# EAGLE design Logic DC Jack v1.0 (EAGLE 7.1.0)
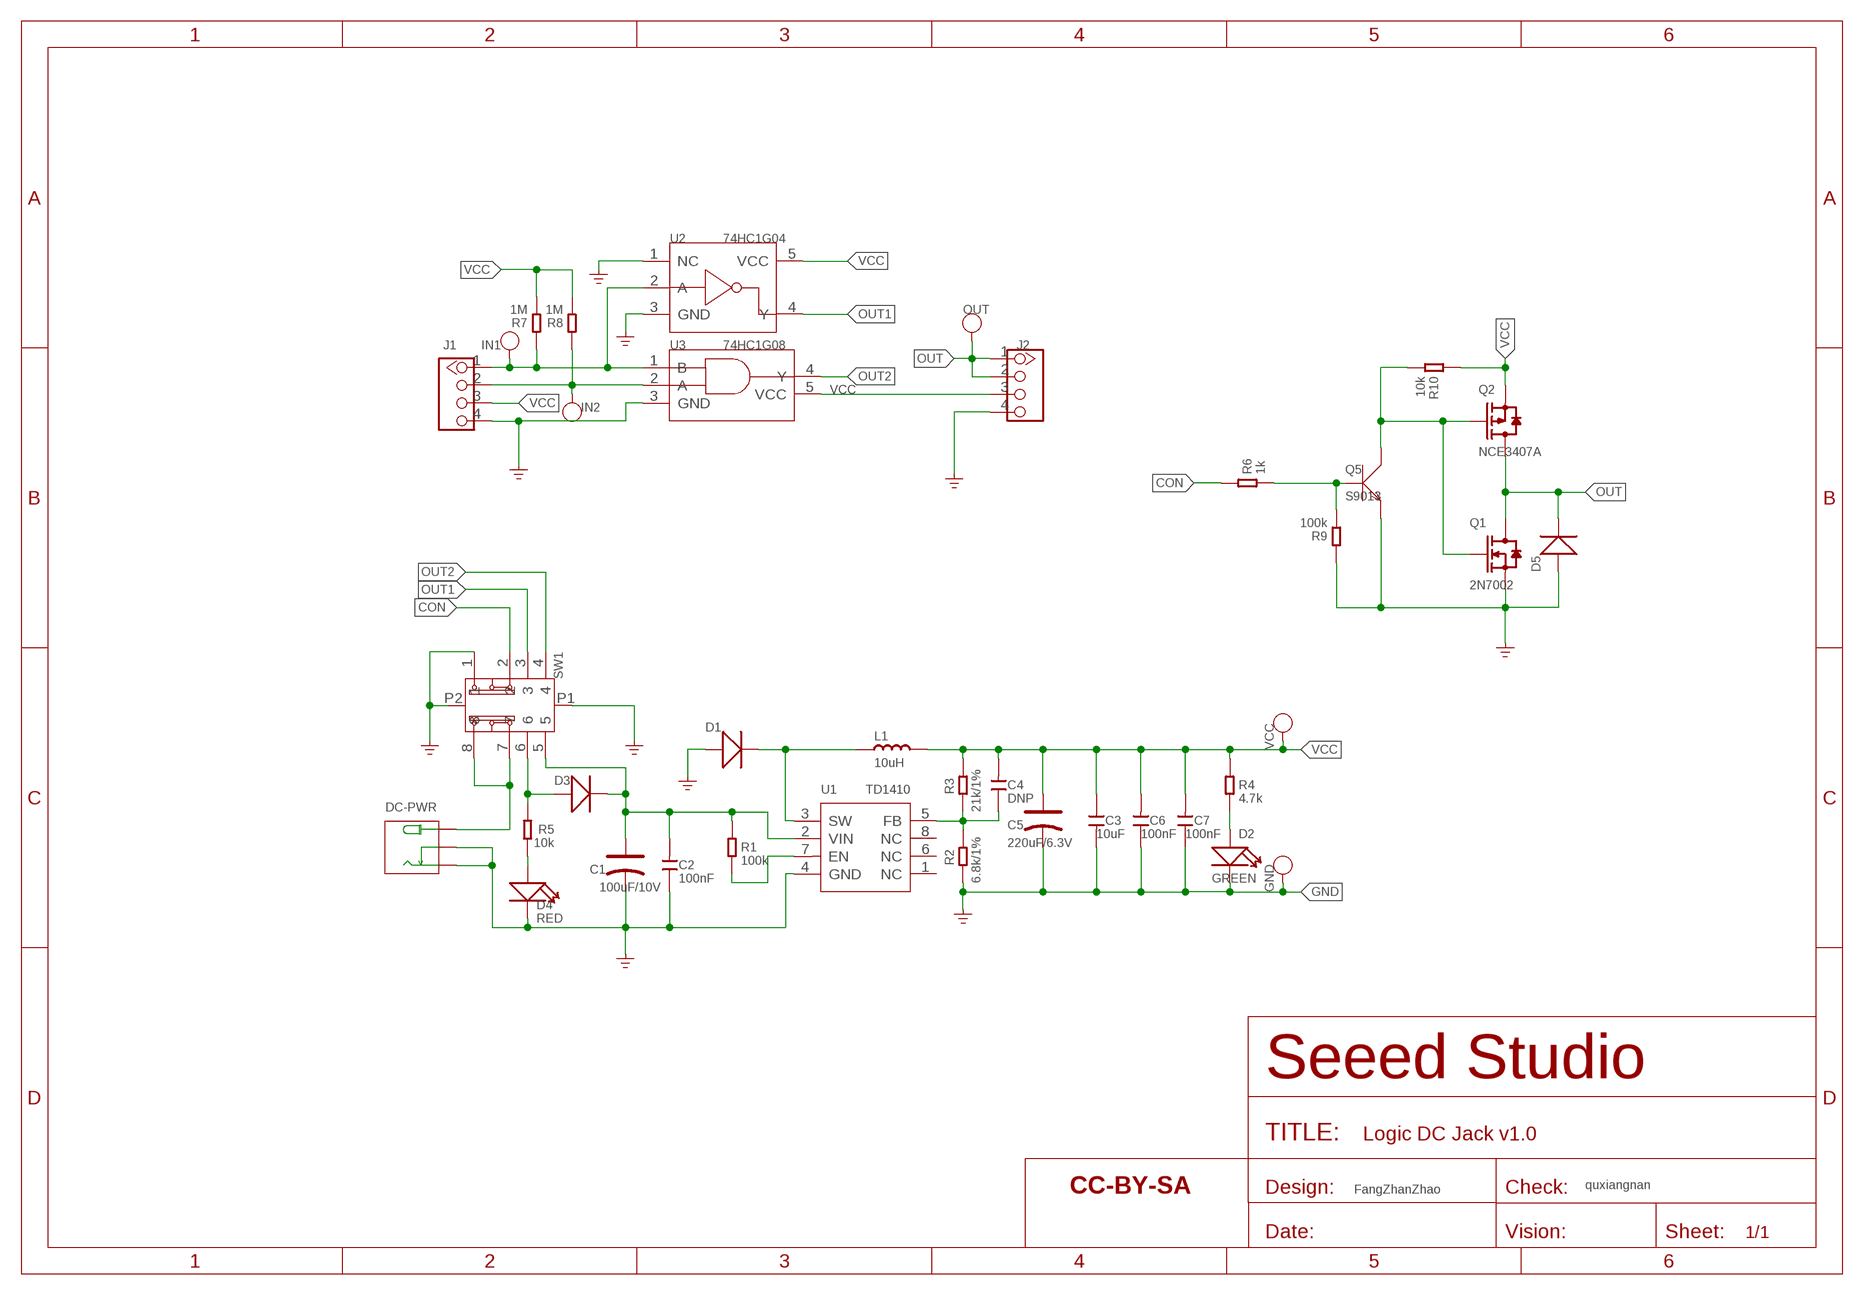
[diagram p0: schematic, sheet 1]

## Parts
C1  100uF/10V  CAP-POLAR-AVX-B  [AVX-B]
C2  100nF  CAP-0603  [C0603]
C3  10uF  CAP-0805  [C0805]
C4  DNP  CAP-0603  [C0603]
C5  220uF/6.3V  CAP-POLAR-AVX-B  [AVX-B]
C6  100nF  CAP-0603  [C0603]
C7  100nF  CAP-0603  [C0603]
D1  DIODE'SMA'  [DO-214AC]
D2  GREEN  LED'0603'  [LED-0603]
D3  304020009  DIODE'SMA'  [DO-214AC]
D4  RED  LED'0603'  [LED-0603]
D5  DIODE'1206'  [SOD-123]
DC-PWR  320120002  POWER-JACK-DC'DC-044'  [3P-L11.6*W9.6*H7.0MM]
GND  PAD-TEST-POINT'4545'  [TP-D45MIL]
IN1  PAD-TEST-POINT'4545'  [TP-D45MIL]
IN2  PAD-TEST-POINT'4545'  [TP-D45MIL]
J1  GROVE-CONNECTOR-DIP-2.0  [4P-2.0]
J2  GROVE-CONNECTOR-DIP-2.0  [4P-2.0]
L1  10uH  INDUCTOR/FERRITE-BEAD'0630'  [L0630]
OUT  PAD-TEST-POINT'4545'  [TP-D45MIL]
Q1  2N7002  MOSFET-N'SOT23'  [SOT-23]
Q2  NCE3407A  MOSFET-P'SI2323CDS/SI2305DS<BR>'  [SOT-23]
Q5  S9013  TRANSISTOR-NPN-SOT23  [SOT-23]
R1  100k  RES-0603  [R0603]
R2  6.8k/1%  RES-0603  [R0603]
R3  21k/1%  RES-0603  [R0603]
R4  4.7k  RES-0603  [R0603]
R5  10k  RES-0603  [R0603]
R6  1k  RES-0603  [R0603]
R7  1M  RES-0603  [R0603]
R8  1M  RES-0603  [R0603]
R9  100k  RES-0603  [R0603]
R10  10k  RES-0603  [R0603]
SW1  SWITCH-SK-23D07SK-22D03H-G4  [8P-3CH-L16*W6.5*H7.5MM-90D]
U1  TD1410  PMIC-TD1410  [SOP-8]
U2  74HC1G04  74HC1G04'GW'  [SOT-353]
U3  74HC1G08  74HC1G08'GW'  [SOT-353]
U$12  SEEEDSTUDIO-OPEN-SCH-FRAME  [SEEEDSTUDIO-PCB-FRAME]
VCC  PAD-TEST-POINT'4545'  [TP-D45MIL]

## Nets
CON: R6.2 SW1.2
GND: C1.- C2.1 C3.2 C5.- C6.1 C7.1 D1.1(+) D2.- D4.- D5.+ DC-PWR.- DC-PWR.CDN GND.T J1.4 J2.4 Q1.2(S) Q5.2(E) R2.1 R9.2 SW1.1 SW1.P1 SW1.P2 U1.4(GND) U2.1(NC) U2.3(GND) U3.3(GND)
N$1: D4.+ R5.1
N$2: C4.1 R2.2 R3.2 U1.5(FB)
N$3: D2.+ R4.1
N$4: D3.1(+) R5.2 SW1.6
N$5: IN1.T J1.1 R7.2 U2.2(A) U3.1(B)
N$6: IN2.T J1.2 R8.2 U3.2(A)
N$7: D1.2(-) L1.1 U1.3(SW)
N$8: DC-PWR.+ SW1.7 SW1.8
N$9: R1.1 U1.7(EN)
N$11: Q5.1(B) R6.1 R9.1
N$12: C1.+ C2.2 D3.2(-) R1.2 SW1.5 U1.2(VIN)
N$13: Q1.1(G) Q2.1(G) Q5.3(C) R10.1
OUT: D5.- J2.1 J2.2 OUT.T Q1.3(D) Q2.3(D)
OUT1: SW1.3 U2.4(Y)
OUT2: SW1.4 U3.4(Y)
VCC: C3.1 C4.2 C5.+ C6.2 C7.2 J1.3 J2.3 L1.2 Q2.2(S) R3.1 R4.2 R7.1 R8.1 R10.2 U2.5(VCC) U3.5(VCC) VCC.T
Unconnected: U1.1(NC) U1.6(NC) U1.8(NC)

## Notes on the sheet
- quxiangnan
- FangZhanZhao

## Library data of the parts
C1 C5 = Discrete-new:CAP-POLAR: Electrolytic Capacitors,Tantalum Capacitors and Super Capacitors
C2-C4 C6 C7 = Discrete-new:CAP: Ceramic Capacitors
D1 D3 D5 = Discrete-new:DIODE*
D2 D4 = Discrete-new:LED
DC-PWR = Connector-new:POWER-JACK-DC: 3P-L11.6*W9.6*H7.0MM:320120002;3P-L14.2*W11.0*H9.0MM:320120003
GND IN1 IN2 OUT VCC = Discrete-new:PAD-TEST-POINT; PARTNO: DNP
J1 J2 = Connector-new:GROVE-CONNECTOR-DIP: 4P-2.0:320110033;4P-2.0-90D:320110034
L1 = Discrete-new:INDUCTOR/FERRITE-BEAD
Q1 = Discrete-new:MOSFET-N: IRLL014: http://www.vishay.com/docs/91319/sihll014.pdf
Q2 = Discrete-new:MOSFET-P
Q5 = Discrete-new:TRANSISTOR-NPN*: NPN audion
R1-R10 = Discrete-new:RES
SW1 = template:SWITCH-SK-23D07
U1 = IC-new:PMIC-TD1410: 310030105
U2 = template:74HC1G04: 74HC1G04 and 74HCT1G04 are high-speed Si-gate CMOS devices. They provide an inverting buffer.
U3 = template:74HC1G08: 2-input AND gate
U$12 = moudle-new:SEEEDSTUDIO-OPEN-SCH-FRAME

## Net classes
0 default: width 0.102 mm, drill 0.203 mm, clearance 0.102 mm
3 usbvcc: width 0.203 mm, drill 0.305 mm, clearance 0.203 mm

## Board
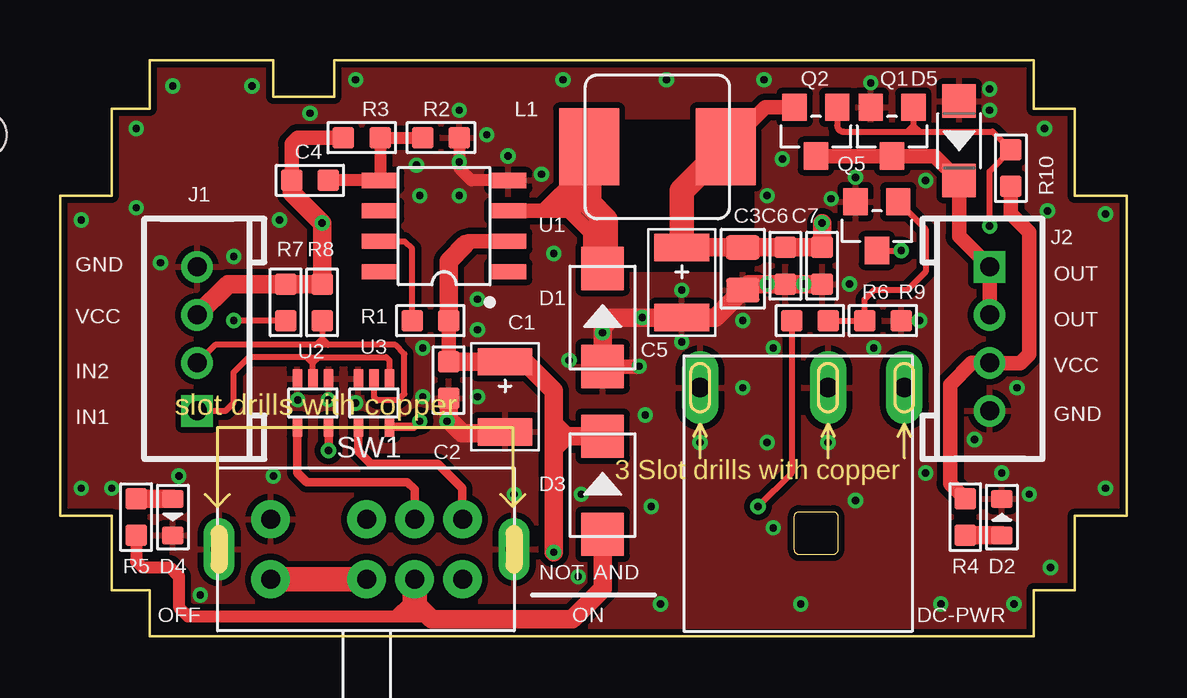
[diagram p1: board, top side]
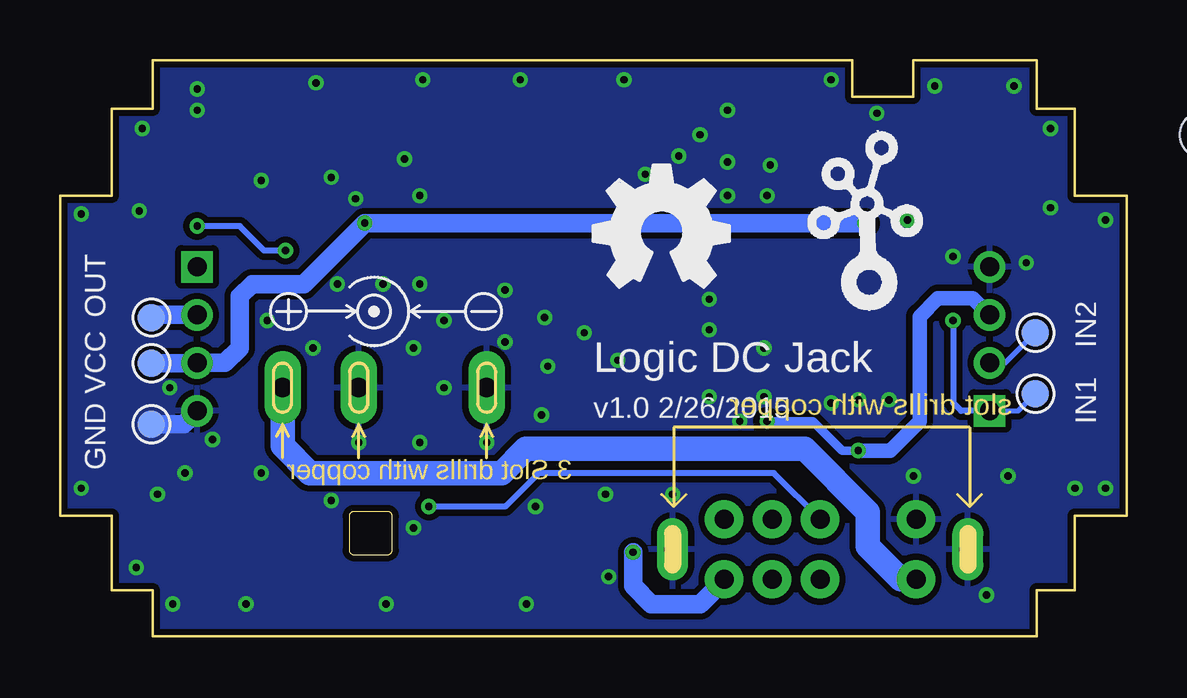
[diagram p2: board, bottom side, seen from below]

Size 44.45 x 24 mm. Coordinates in mm from the lower left corner, seen from the top.
Outline: 3.75,1.9 3.75,0 40.58,0 40.58,1.9 42.29,1.9 42.29,5.02 44.45,5.02 44.45,18.35 42.29,18.35 42.29,21.97 40.58,21.97 40.58,24 11.43,24 11.43,22.48 8.89,22.48 8.89,24 3.75,24 3.75,21.97 2.16,21.97 2.16,18.35 0,18.35 0,5.02 2.16,5.02 2.16,1.9 3.75,1.9
Copper layers (1*16): Top 0.035mm / dielectric 1.5mm / Bottom 0.035mm
Design rules "SeeedStudio_2layer_DRU_no_angle_20140221 *": minimum track width 4mil, minimum drill 10mil, track to track 8mil, track to pad 8mil, pad to pad 8mil, via to via 6mil, smd to smd 0mil, copper to edge 10mil, drill to drill 10mil, minimum pad ring 10mil, minimum via ring 6mil, stop-mask expansion 2mil, vias tented up to drill 25mil, thermal gap 10mil
Holes 1.91 mm at -3.17,20.89 136.53,20.89 -3.17,-139.13 136.53,-139.13
tRestrict: area 22.9,15.4 to 28.7,21.3

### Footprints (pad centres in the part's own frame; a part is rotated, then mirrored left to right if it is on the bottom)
AVX-B = smd 1.143 x 2.286: + -1.46,0; - 1.46,0
C0603 = smd 0.889 x 0.889: 1 -0.762,0; 2 0.762,0
C0805 = smd 1.016 x 1.397: 1 -0.889,0; 2 0.889,0
DO-214AC = smd 1.8 x 1.77: 1 -2.042,0; 2 2.042,0
LED-0603 = smd 0.762 x 0.889: + -0.762,0; - 0.762,0
SOD-123 = smd 1.397 x 1.397: + -1.651,0; - 1.651,0
3P-L11.6*W9.6*H7.0MM = drill 0.813 pad 1.524 long: + 4.381,10.16; - -4.128,10.16; CDN 1.206,10.16
TP-D45MIL = smd 1.143 x 1.143: T 0,0
4P-2.0 = drill 0.8 pad 1.27 square: 1 -3,0 | drill 0.8 pad 1.27: 2 -1,0; 3 1,0; 4 3,0
L0630 = smd 2.5 x 3.2: 1 -2.85,0; 2 2.85,0
SOT-23 = smd 1.016 x 1.143: 1 -0.889,-1.016; 2 0.889,-1.016; 3 0,1.016
R0603 = smd 0.889 x 0.889: 1 -0.762,0; 2 0.762,0
8P-3CH-L16*W6.5*H7.5MM-90D = drill 0.8 pad 1.6: 1 -4,1.25; 2 0,1.25; 3 2,1.25; 4 4,1.25; 5 4,-1.25; 6 2,-1.25; 7 0,-1.25; 8 -4,-1.25 | drill 0.7 pad 1.3 long: P1 -6.15,0; P2 6.15,0
SOP-8 = smd 0.635 x 1.524: 1 -1.905,-2.667; 2 -0.635,-2.667; 3 0.635,-2.667; 4 1.905,-2.667; 5 1.905,2.667; 6 0.635,2.667; 7 -0.635,2.667; 8 -1.905,2.667
SOT-353 = smd 0.4 x 0.8: 1 -0.65,-1; 2 0,-1; 3 0.65,-1; 4 0.65,1; 5 -0.65,1

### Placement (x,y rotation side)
C1  18.54,9.97 270 top
C2  16.19,10.67 90 top
C3  28.45,15.3 270 top
C4  10.41,18.99 180 top
C5  25.91,14.73 270 top
C6  30.23,15.43 90 top
C7  31.75,15.43 90 top
D1  22.61,13.27 90 top
D2  39.24,4.95 90 top
D3  22.61,6.29 90 top
D4  4.7,4.95 270 top
D5  37.47,20.64 270 top
DC-PWR  30.8,0.19 0 top
GND  40.64,8.83 0 bottom
IN1  3.81,10.1 0 bottom
IN2  3.81,12.64 0 bottom
J1  5.71,12.38 90 top
J2  38.73,12.38 270 top
L1  24.89,20.38 0 top
OUT  40.64,13.27 0 bottom
Q1  34.67,21.02 180 top
Q2  31.5,21.02 180 top
Q5  34.04,17.08 180 top
R1  15.43,13.14 0 top
R2  15.88,20.76 180 top
R3  12.57,20.76 0 top
R4  37.72,4.95 90 top
R5  3.18,4.95 270 top
R6  31.24,13.14 180 top
R7  9.4,13.91 270 top
R8  10.92,13.91 270 top
R9  34.29,13.14 0 top
R10  39.62,19.49 270 top
SW1  12.78,3.62 0 top
U1  16,17.08 90 top
U2  10.54,9.72 180 top
U3  13.08,9.72 180 top
U$1  [OSHW_FILLX200_NOTEXT]  22.23,14.54 0 bottom
U$11  [GROVE-SILK-BIG]  10.8,14.54 0 bottom
U$12  not placed on the board
VCC  40.64,11.37 0 bottom

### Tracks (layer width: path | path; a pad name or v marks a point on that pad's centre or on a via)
CON  (via drill 0.3 pad 0.64)
  Top 0.254: R6.2 30.48,6.79 v29.08,5.4
  Bottom 0.254: v29.08,5.4 25.91,5.4 24.51,6.79 14.7,6.79 SW1.2
GND  (via drill 0.3 pad 0.64)
  Top 0.508: R2.1 16.64,19.49 17.15,18.99 U1.4
  Top 0.61: D1.1 24.12,11.23 v24.13,11.24
  Top 0.762: C2.1 16.19,9.02 16.76,8.45 18.48,8.45 C1.- | C7.1 C6.1 28.7,14.67 C3.2 27.3,13.27 C5.- 22.99,13.27 22.61,12.89 D1.1
  Bottom 0.762: GND.T 39.29,8.83 J2.4
  other vias: 28.45,13.14 24.26,13.27 22.61,12.64 21.21,11.49 32.89,14.67 29.46,14.67 30.99,14.67 33.91,12 35.81,13.14 32.13,18.22 33.78,23.05 38.73,21.91 38.73,22.8 18.67,20 16.64,21.91 17.78,20.89 16.64,19.75 9.91,9.84 12.32,9.72 11.18,9.84 33.15,19.11 40.39,5.91 39.24,6.79 4.7,22.92 8,22.92 12.32,23.18 20.96,23.18 29.34,23.18 41.02,21.15 43.56,17.59 43.56,6.16 41.28,2.86 39.75,1.33 25.02,1.33 30.86,1.33 36.7,1.33 21.72,5.91 24.64,5.4 26.67,8.06 3.18,21.15 3.18,17.84 0.89,17.34 0.89,6.16 2.16,6.16 5.84,1.71 4.95,6.67 4.19,15.56 9.14,17.34 10.41,21.78 25.27,23.18 30.1,19.88 29.46,18.35 20.07,19.24 20.57,15.94 25.91,14.41 25.91,12.26 28.45,10.35 32,8.06 21.59,2.48 36.07,6.79 36.07,18.99 8.89,6.67 29.72,4.51 29.46,8.06 29.72,12 33.15,5.65 38.1,8.19 39.88,10.35 41.15,17.72 7.24,15.81 14.86,19.62 14.99,18.35 16.64,18.35 17.4,14.03 17.4,12.76 16.13,8.95 17.4,9.97 15.11,9.97 15.11,12 18.92,5.91 24.38,9.21
  pour Top (isolate 0.254): -3.68,27.37 46.48,27.37 46.48,-5.02 -3.68,-5.02
  pour Bottom (isolate 0.254): -3.68,27.75 46.48,27.75 46.48,-4.64 -3.68,-4.64
N$1
  Top 0.762: R5.1 D4.+
N$2
  Top 0.508: R2.2 R3.2 U1.5 C4.1
N$3
  Top 0.762: R4.1 D2.+
N$4
  Top 0.508: R5.2 3.18,3.11 3.43,2.86 4.57,2.86 4.95,2.48 4.95,1.21 5.33,0.83 13.97,0.83 | 13.97,0.83 14.19,0.83 | 14.19,0.83 14.38,1.02 | 14.38,1.02 14.78,1.42 | 14.38,1.02 15.17,1.02 15.24,0.95 | 14.19,0.83 15.37,0.83 15.49,0.7 | 13.97,0.83 14.61,1.46
  Top 0.762: 14.78,1.42 15.24,0.95 15.49,0.7 21.34,0.7 22.61,1.97 D3.1
  Top 1.016: 14.78,1.42 SW1.6
N$5  (via drill 0.3 pad 0.64)
  Top 0.254: R7.2 v7.24,13.14 | U2.2 10.54,11.37 | 10.54,11.37 10.29,11.62 | 10.29,11.62 10.8,11.62 | 10.54,11.37 10.8,11.62 | 10.8,11.62 13.59,11.62 13.73,11.48 U3.1 | 10.29,11.62 7.87,11.62 7.24,10.99 7.24,9.72 6.91,9.38 J1.1
  Bottom 0.203: J1.1 4.52,9.38 IN1.T
  Bottom 0.254: v7.24,13.14 7.24,9.72 6.91,9.38 J1.1
N$6
  Top 0.254: R8.2 10.92,12.38 | 10.92,12.38 10.67,12.13 | U3.2 13.08,9.97 13.21,9.84 14.1,9.84 14.35,10.1 14.35,11.75 13.97,12.13 11.18,12.13 | 11.18,12.13 10.67,12.13 | 10.92,12.38 11.18,12.13 | 10.67,12.13 6.46,12.13 J1.2
  Bottom 0.203: J1.2 5.06,11.38 IN2.T
N$7
  Top 0.61: 21.46,19.04 20.26,17.84 21.08,17.84 22.1,16.83 22.1,15.05 22.23,14.92 | 21.46,19.04 21.56,19.14 | 21.56,19.14 22.04,19.62 | 21.46,19.04 21.46,18.1 | 21.46,18.1 21.46,17.84 21.08,18.22 21.08,18.61 21.59,19.11 21.57,19.14 21.56,19.14 | U1.3 21.08,17.72 21.46,18.1
  Top 1.016: L1.1 22.04,19.62 22.04,18.03 22.73,17.34 22.73,15.44 D1.2
N$8
  Top 1.016: SW1.7 SW1.8
  Bottom 1.016: SW1.8 9.42,2.37 10.8,3.75 10.8,5.17 13.42,7.8 | DC-PWR.+ 35.18,7.94 34.04,6.79 26.04,6.79 25.03,7.8 13.42,7.8 | 13.42,7.8
N$9
  Top 0.254: U1.7 14.35,16.45 14.67,16.13 R1.1
N$11
  Top 0.254: R6.1 R9.1 33.53,14.03 33.91,14.41 35.31,14.41 36.07,15.18 36.07,16.95 Q5.1
N$12  (via drill 0.3 pad 0.64)
  Top 0.61: C2.2 R1.2 | 16.32,15.75 16.89,16.32 17.02,16.45 U1.2
  Top 0.762: 19.11,11.43 C1.+ C2.2 | 19.11,11.43 19.18,11.49 | 19.11,11.43 19.37,11.43 20.57,10.22 20.57,8.83 | 20.57,8.83 21.08,8.32 | 21.08,8.32 22.6,8.32 D3.2 | R1.2 16.19,15.62 16.89,16.32 | 20.57,8.83 v20.57,3.49 | 21.08,8.32 20.7,7.94
  Bottom 0.762: 16.78,2.34 17.78,1.33 19.81,1.33 20.57,2.1 v20.57,3.49
  Bottom 1.016: 16.78,2.34 SW1.5
N$13  (via drill 0.3 pad 0.64)
  Top 0.254: Q5.3 v35.05,16.07 | v38.73,17.08 38.73,19.37 R10.1 38.86,21.02 35.81,21.02 | Q2.1 32.39,21.27 arc90 32.64,21.02 35.31,21.02 | 35.31,21.02 35.56,21.02 | 35.56,21.02 35.81,21.02 | Q1.1 35.56,21.27 | 35.56,21.27 35.56,21.02 | 35.56,21.27 35.31,21.02 | 35.56,21.27 35.81,21.02
  Bottom 0.254: v35.05,16.07 35.94,16.07 36.96,17.08 v38.73,17.08
OUT
  Top 0.61: Q2.3 Q1.3 36.45,20 D5.- 37.47,16.65 J2.1 J2.2
  Bottom 0.762: J2.2 40.53,13.38 OUT.T
OUT1
  Top 0.356: U2.4 9.89,6.81 10.29,6.41 14.48,6.41 14.78,6.12 SW1.3
OUT2
  Top 0.356: U3.4 12.43,7.7 12.95,7.18 15.75,7.18 16.76,6.16 16.76,4.88 SW1.4
VCC  (via drill 0.3 pad 0.64)
  Top 0.356: U2.5 v11.19,7.73 | U3.5 14.75,8.72 v14.99,8.95
  Top 0.61: R10.2 39.62,17.59 40.39,16.83 40.39,11.75 40.01,11.37 38.75,11.37 J2.3 37.99,11.38 37.08,10.48 37.08,6.35 R4.2 | Q2.2 29.39,22.03 L1.2 | R3.1 9.91,20.76 9.65,20.51 C4.2
  Top 0.762: C5.+ C3.1 C6.2 C7.2 v31.75,17.21 | C4.2 9.65,18.48 v10.92,17.21 R8.1 R7.1 7,14.67 J1.3
  Top 1.016: C5.+ 25.91,18.55 L1.2
  Bottom 0.356: v14.99,8.95 13.08,8.95 11.86,7.73 v11.19,7.73
  Bottom 0.61: v11.19,7.73 9.86,7.73 8.64,8.96 8.64,13.31 7.87,14.08 | J1.3 6.41,14.08 7.87,14.08 | 7.87,14.08
  Bottom 0.762: v10.92,17.21 v31.75,17.21 34.29,14.67 36.45,14.67 36.96,14.16 36.96,12 37.58,11.38 J2.3 38.75,11.37 VCC.T

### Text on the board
tPlace: GND | OUT | VCC | OUT | IN2 | VCC | IN1 | GND | NOT | AND | OFF | ON
bPlace: Logic DC Jack | v1.0 2/26/2015

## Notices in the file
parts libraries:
moudle-new: This work is licensed under the Creative Commons Attribution 4.0 International License.
To view a copy of this license,visit:
http://creativecommons.org/licenses/by-sa/4.0
moudle-new: CC-BY-SA
